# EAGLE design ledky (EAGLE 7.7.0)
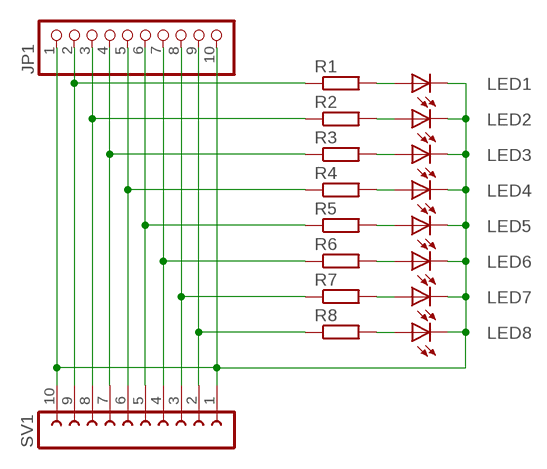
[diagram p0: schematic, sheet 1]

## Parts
JP1  PINHD-1X10  [1X10]
LED1  LED3MM  [LED3MM]
LED2  LED3MM  [LED3MM]
LED3  LED3MM  [LED3MM]
LED4  LED3MM  [LED3MM]
LED5  LED3MM  [LED3MM]
LED6  LED3MM  [LED3MM]
LED7  LED3MM  [LED3MM]
LED8  LED3MM  [LED3MM]
R1  R-EU_0207/10  [0207/10]
R2  R-EU_0207/10  [0207/10]
R3  R-EU_0207/10  [0207/10]
R4  R-EU_0207/10  [0207/10]
R5  R-EU_0207/10  [0207/10]
R6  R-EU_0207/10  [0207/10]
R7  R-EU_0207/10  [0207/10]
R8  R-EU_0207/10  [0207/10]
SV1  FE10-1  [FE10]

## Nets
N$1: LED1.A R1.2
N$2: JP1.1 JP1.10 LED1.K(C) LED2.K(C) LED3.K(C) LED4.K(C) LED5.K(C) LED6.K(C) LED7.K(C) LED8.K(C) SV1.1 SV1.10
N$3: JP1.9 R8.1 SV1.2
N$4: JP1.8 R7.1 SV1.3
N$5: JP1.7 R6.1 SV1.4
N$6: JP1.6 R5.1 SV1.5
N$7: JP1.5 R4.1 SV1.6
N$8: JP1.4 R3.1 SV1.7
N$9: JP1.3 R2.1 SV1.8
N$10: JP1.2 R1.1 SV1.9
N$11: LED2.A R2.2
N$12: LED3.A R3.2
N$13: LED4.A R4.2
N$14: LED5.A R5.2
N$15: LED6.A R6.2
N$16: LED7.A R7.2
N$17: LED8.A R8.2

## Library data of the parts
JP1 = pinhead:PINHD-1X10: PIN HEADER
LED1-LED8 = led:LED: LED
R1-R8 = resistor:R-EU_: RESISTOR, European symbol
SV1 = con-lsta:FE10-1: FEMALE HEADER; OC_FARNELL: unknown; OC_NEWARK: unknown

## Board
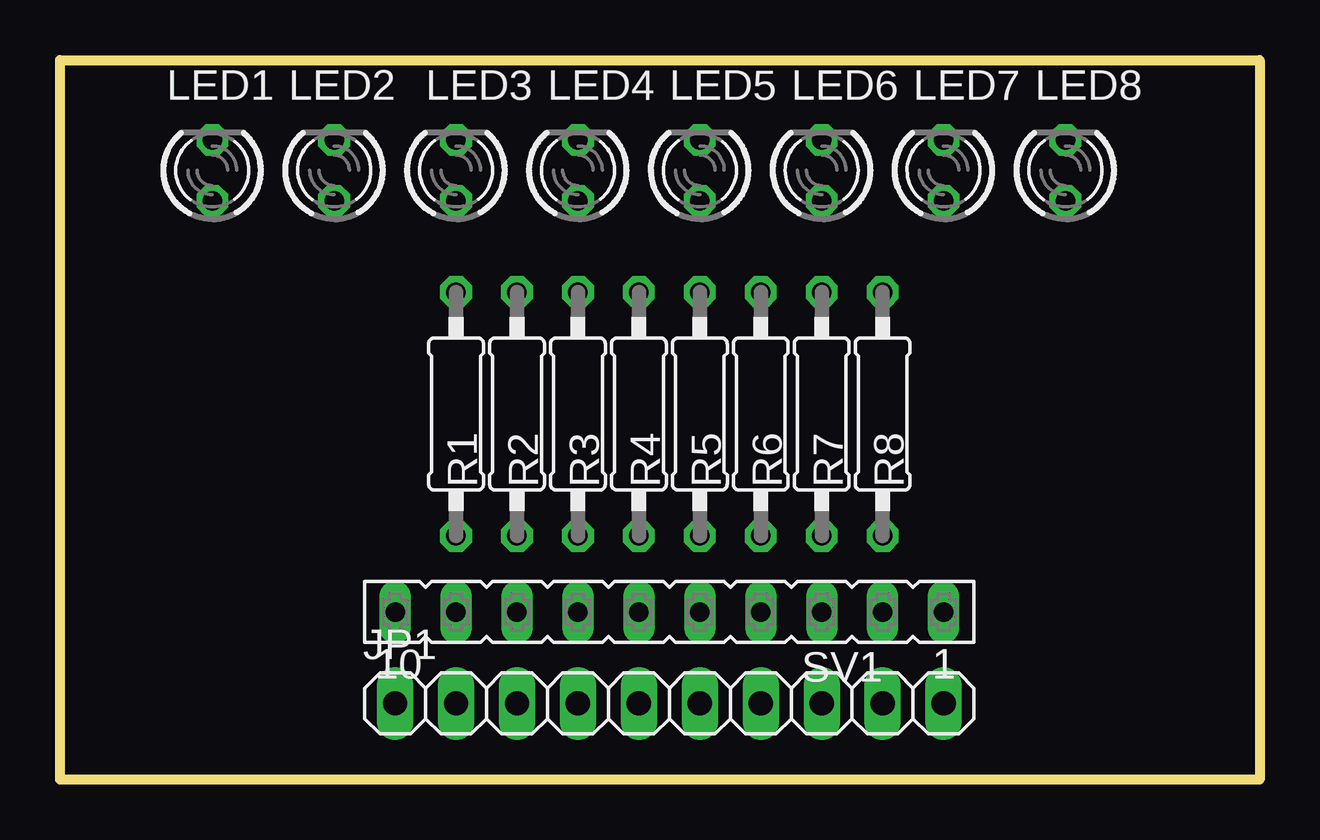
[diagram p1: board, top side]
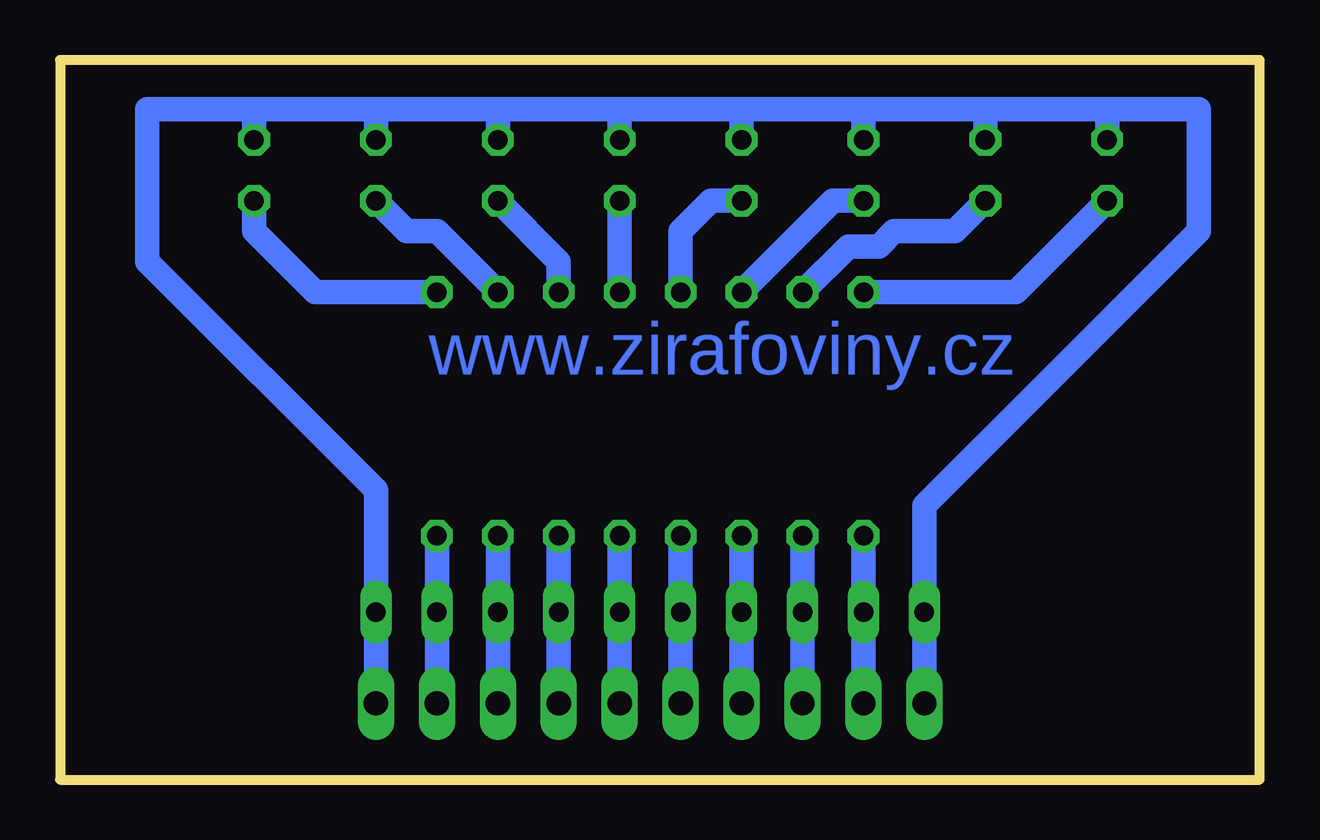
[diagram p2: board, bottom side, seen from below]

Size 50 x 30 mm. Coordinates in mm from the lower left corner, seen from the top.
Outline: 0,0 0,30 50,30 50,0 0,0
Copper layers (1*16): Top 0.035mm / dielectric 1.5mm / Bottom 0.035mm
Design rules "default": minimum track width 10mil, minimum drill 24mil, track to track 8mil, track to pad 8mil, pad to pad 8mil, via to via 8mil, smd to smd 8mil, copper to edge 40mil, drill to drill 8mil, minimum pad ring 10mil, minimum via ring 8mil, stop-mask expansion 4mil, vias tented up to drill 0mil, thermal gap 10mil

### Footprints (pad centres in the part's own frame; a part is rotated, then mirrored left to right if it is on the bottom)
1X10 = drill 1.016 long: 1 -11.43,0; 2 -8.89,0; 3 -6.35,0; 4 -3.81,0; 5 -1.27,0; 6 1.27,0; 7 3.81,0; 8 6.35,0; 9 8.89,0; 10 11.43,0
LED3MM = drill 0.813 octagon: A -1.27,0; K 1.27,0
0207/10 = drill 0.813 octagon: 1 -5.08,0; 2 5.08,0
FE10 = drill 0.813 long: 1 -11.43,0; 2 -8.89,0; 3 -6.35,0; 4 -3.81,0; 5 -1.27,0; 6 1.27,0; 7 3.81,0; 8 6.35,0; 9 8.89,0; 10 11.43,0

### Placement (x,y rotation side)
JP1  25.4,3.17 0 top
LED1  6.35,25.4 90 top
LED2  11.43,25.4 90 top
LED3  16.51,25.4 90 top
LED4  21.59,25.4 90 top
LED5  26.67,25.4 90 top
LED6  31.75,25.4 90 top
LED7  36.83,25.4 90 top
LED8  41.91,25.4 90 top
R1  16.51,15.24 90 top
R2  19.05,15.24 90 top
R3  21.59,15.24 90 top
R4  24.13,15.24 90 top
R5  26.67,15.24 90 top
R6  29.21,15.24 90 top
R7  31.75,15.24 90 top
R8  34.29,15.24 90 top
SV1  25.4,6.99 180 top

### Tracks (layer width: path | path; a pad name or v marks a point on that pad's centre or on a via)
N$1
  Bottom 1.016: R1.2 10.16,20.32 LED1.A
N$2
  Bottom 1.016: LED1.K 6.35,27.94 | 6.35,27.94 11.43,27.94 | 11.43,27.94 16.51,27.94 | 16.51,27.94 21.59,27.94 | 21.59,27.94 26.67,27.94 | 26.67,27.94 31.75,27.94 | 31.75,27.94 36.83,27.94 | 36.83,27.94 41.91,27.94 | 41.91,27.94 LED8.K | LED7.K 36.83,27.94 | LED6.K 31.75,27.94 | LED5.K 26.67,27.94 | LED4.K 21.59,27.94 | LED3.K 16.51,27.94 | LED2.K 11.43,27.94 | JP1.1 SV1.10 13.97,11.43 2.54,22.86 2.54,27.94 6.35,27.94 | SV1.1 JP1.10 36.83,12.06 46.35,21.59 46.35,27.94 41.91,27.94
N$3
  Bottom 1.016: JP1.9 SV1.2 R8.1
N$4
  Bottom 1.016: JP1.8 SV1.3 R7.1
N$5
  Bottom 1.016: JP1.7 SV1.4 R6.1
N$6
  Bottom 1.016: JP1.6 SV1.5 R5.1
N$7
  Bottom 1.016: JP1.5 SV1.6 R4.1
N$8
  Bottom 1.016: JP1.4 SV1.7 R3.1
N$9
  Bottom 1.016: JP1.3 SV1.8 R2.1
N$10
  Bottom 1.016: JP1.2 SV1.9 R1.1
N$11
  Bottom 1.016: R2.2 17.14,22.23 15.88,22.23 15.24,22.86 12.7,22.86 LED2.A
N$12
  Bottom 1.016: R3.2 17.78,24.13 LED3.A
N$13
  Bottom 1.016: R4.2 24.13,22.86 22.86,24.13 LED4.A
N$14
  Bottom 1.016: R5.2 LED5.A
N$15
  Bottom 1.016: R6.2 29.21,21.59 LED6.A
N$16
  Bottom 1.016: R7.2 34.29,22.86 35.56,22.86 LED7.A
N$17
  Bottom 1.016: LED8.A 41.91,22.86 39.37,20.32 R8.2

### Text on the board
Bottom: www.zirafoviny.cz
